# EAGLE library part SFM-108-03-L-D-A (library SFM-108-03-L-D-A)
.050" Tiger Eye High-Reliability Socket Strip, pos per row Source: Datasheet
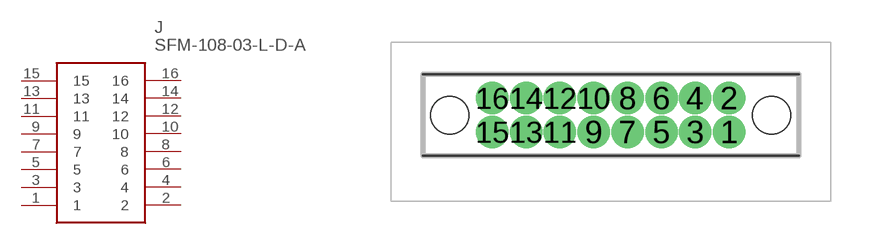
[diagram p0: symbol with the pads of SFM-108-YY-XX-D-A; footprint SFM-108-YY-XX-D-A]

Designator prefix J

## SFM-108-03-L-D-A (Description: .050" Tiger Eye High-Reliability Socket Strip, pos per row; Height: mm; Manufacturer_Name: SAMTEC; Manufacturer_Part_Number: SFM-108-03-L-D-A)  [SFM-108-YY-XX-D-A]
1  1
2  2
3  3
4  4
5  5
6  6
7  7
8  8
9  9
10  10
11  11
12  12
13  13
14  14
15  15
16  16

## Footprint SFM-108-YY-XX-D-A (pad centres in mm)
SFM-108-YY-XX-D-A
drill 0.71 pad 1.1: 1 0,0; 2 0,1.27; 3 -1.27,0; 4 -1.27,1.27; 5 -2.54,0; 6 -2.54,1.27; 7 -3.81,0; 8 -3.81,1.27; 9 -5.08,0; 10 -5.08,1.27; 11 -6.35,0; 12 -6.35,1.27; 13 -7.62,0; 14 -7.62,1.27; 15 -8.89,0; 16 -8.89,1.27
hole 1.42 at 1.59,0.635
hole 1.42 at -10.48,0.635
